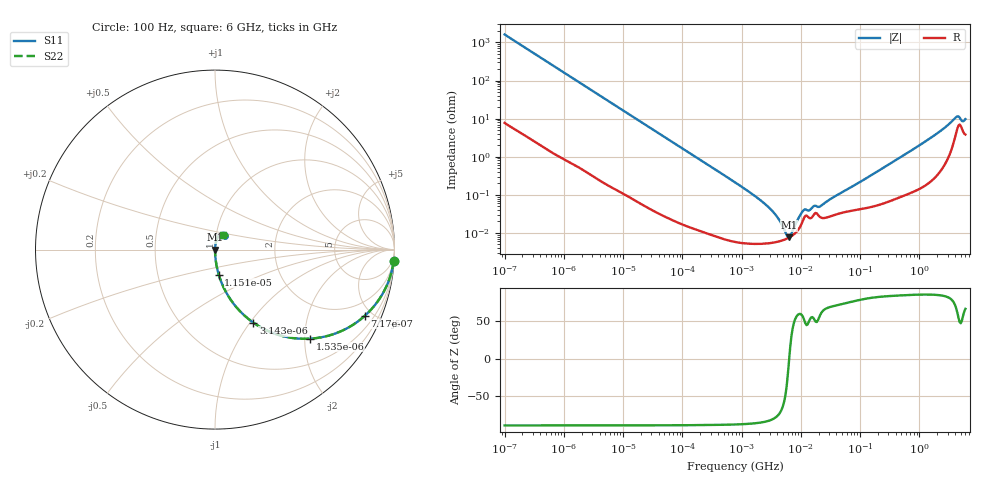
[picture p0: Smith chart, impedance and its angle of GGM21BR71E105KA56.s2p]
!Murata Part Number: GGM21BR71E105KA56
!These Parameters are Measured in Series Mode Connection
!Data Generated on Mar 13, 2026
!  o--ll--o
!Port1  Port2
!  o------o
!Operation Temp=25[degC], DC Bias Voltage=0[V]
!Freq. Start=100[Hz] Stop=6[GHz] 401[Steps]
# Hz S RI R 50
!Freq.(Hz) S11(Real) S11(Imag) S21(Real) S21(Imag) S12(Real) S12(Imag) S22(Real) S22(Imag)
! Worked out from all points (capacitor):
!   401 points, 100 Hz to 6 GHz, reference 50 ohm
!   read as one part in series: C = 984 nF near 109 Hz
!   lowest |Z| = 7.61 mohm at 6.353 MHz (marker M1)
!   series resonance near 6.361 MHz, so ESL is about 640 pH
!   S11 on the Smith chart (normalised r, x): 100 Hz: 1, -32; 717 Hz: 1.02, -4.53; 1.535 kHz: 1.01, -2.12; 3.143 kHz: 1.01, -1.04; 11.51 kHz: 1.00, -0.29; 6 GHz: 1.08, +0.18
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100  0.9959 -0.0616  0.00411 0.0616  0.00411 0.0616  0.9959 -0.0616
335  0.9582 -0.1977  0.0418 0.1977  0.0418 0.1977  0.9582 -0.1977
717  0.8358 -0.368  0.1642 0.368  0.1642 0.368  0.8358 -0.368
1535  0.5295 -0.4963  0.4705 0.4963  0.4705 0.4963  0.5295 -0.4963
2008  0.398 -0.4866  0.602 0.4866  0.602 0.4866  0.398 -0.4866
3143  0.2141 -0.4073  0.7859 0.4073  0.7859 0.4073  0.2141 -0.4073
5625  0.0795 -0.2675  0.9205 0.2675  0.9205 0.2675  0.0795 -0.2675
11514  0.0208 -0.1395  0.9792 0.1395  0.9792 0.1395  0.0208 -0.1395
40335  0.00199 -0.0408  0.998 0.0408  0.998 0.0408  0.00199 -0.0408
774597  6.26e-05 -0.00213  0.9999 0.00213  0.9999 0.00213  6.26e-05 -0.00213
2837864  5.37e-05 -0.000475  0.9999 0.000475  0.9999 0.000475  5.37e-05 -0.000475
4060267  5.88e-05 -0.000247  0.9999 0.000247  0.9999 0.000247  5.88e-05 -0.000247
5554849  6.88e-05 -7.31e-05  0.9999 7.31e-05  0.9999 7.31e-05  6.88e-05 -7.31e-05
6353432  7.61e-05 -6e-07  0.9999 6e-07  0.9999 6e-07  7.61e-05 -6e-07
7266822  8.68e-05 7.33e-05  0.9999 -7.33e-05  0.9999 -7.33e-05  8.68e-05 7.33e-05
1.087309e7  0.000212 0.000314  0.9998 -0.000314  0.9998 -0.000314  0.000212 0.000314
1.555665e7  0.00026 0.000382  0.9997 -0.000382  0.9997 -0.000382  0.00026 0.000382
2.225763e7  0.00025 0.000461  0.9997 -0.000461  0.9997 -0.000461  0.00025 0.000461
3.124326e8  0.000714 0.00637  0.9993 -0.00637  0.9993 -0.00637  0.000714 0.00637
1.712697e9  0.00371 0.0343  0.9963 -0.0343  0.9963 -0.0343  0.00371 0.0343
4.193612e9  0.0494 0.0928  0.9506 -0.0928  0.9506 -0.0928  0.0494 0.0928
6e9  0.044 0.0823  0.956 -0.0823  0.956 -0.0823  0.044 0.0823
